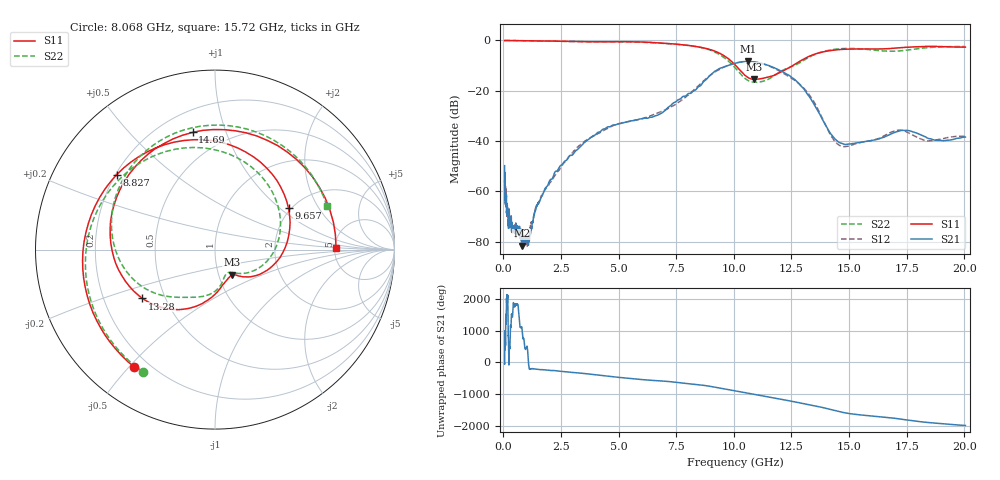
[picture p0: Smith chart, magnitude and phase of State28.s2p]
# Hz S DB R 50
!freq MagS11 AngS11 MagS21 AngS21 MagS12 AngS12 MagS22 AngS22
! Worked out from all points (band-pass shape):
!   1601 points, 50 MHz to 20.05 GHz, reference 50 ohm
!   highest |S21| = -8.33 dB at 10.61 GHz (marker M1); lowest = -81.6 dB at 796.7 MHz (marker M2)
!   |S21| within 3 dB of the highest: 9.338 GHz to 11.86 GHz (2.519 GHz wide, 23.8 % of centre)
!   lowest |S11| = -15.5 dB at 10.89 GHz (marker M3), VSWR 1.40, Z = 57.7 - j16.7 ohm
!   |S11| at or under -10 dB: 10.09 GHz to 12.55 GHz (2.463 GHz wide, 21.8 % of centre)
!   |S22| runs from -16.6 to 0.0 dB; largest |S21 - S12| = 0.014
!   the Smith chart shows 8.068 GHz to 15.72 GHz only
!   S11 on the Smith chart (normalised r, x): 8.068 GHz: 0.15, -0.51; 8.827 GHz: 0.20, +0.33; 9.657 GHz: 1.94, +1.15; 13.28 GHz: 0.37, -0.27; 14.69 GHz: 0.33, +0.77; 15.72 GHz: 5.14, +0.17
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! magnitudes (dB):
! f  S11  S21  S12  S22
! 50 MHz  0.0  -49.8  -56.6  0.0
! 87.05 MHz  0.0  -63.8  -58.6  0.0
! 124.3 MHz  0.0  -62.5  -62.2  0.0
! 135.9 MHz  0.0  -68.1  -65.1  0.0
! 227.1 MHz  0.0  -72.2  -74.2  0.0
! 246.6 MHz  0.0  -67.4  -73.7  0.0
! 334.1 MHz  0.0  -72.7  -70.3  0.0
! 369.6 MHz  0.0  -72.8  -75.0  0.0
! 796.7 MHz  -0.1  -81.6  -78.1  -0.1
! 1.005 GHz  -0.1  -77.8  -80.5  -0.1
! 1.104 GHz  -0.1  -79.2  -78.9  -0.1
! 2.722 GHz  -0.3  -47.7  -47.6  -0.4
! 7.402 GHz  -1.4  -24.7  -25.7  -1.4
! 8.068 GHz  -2.0  -21.1  -21.3  -2.0
! 8.827 GHz  -3.2  -15.3  -15.0  -3.4
! 9.657 GHz  -6.6  -10.2  -10.2  -7.4
! 10.61 GHz  -14.7  -8.3  -8.4  -15.9
! 10.89 GHz  -15.5  -8.5  -8.6  -16.6
! 13.28 GHz  -6.2  -22.4  -21.7  -6.6
! 14.69 GHz  -3.5  -41.0  -42.1  -3.2
! 15.72 GHz  -3.4  -40.2  -40.2  -3.5
! 20.05 GHz  -2.7  -38.4  -38.1  -2.4
